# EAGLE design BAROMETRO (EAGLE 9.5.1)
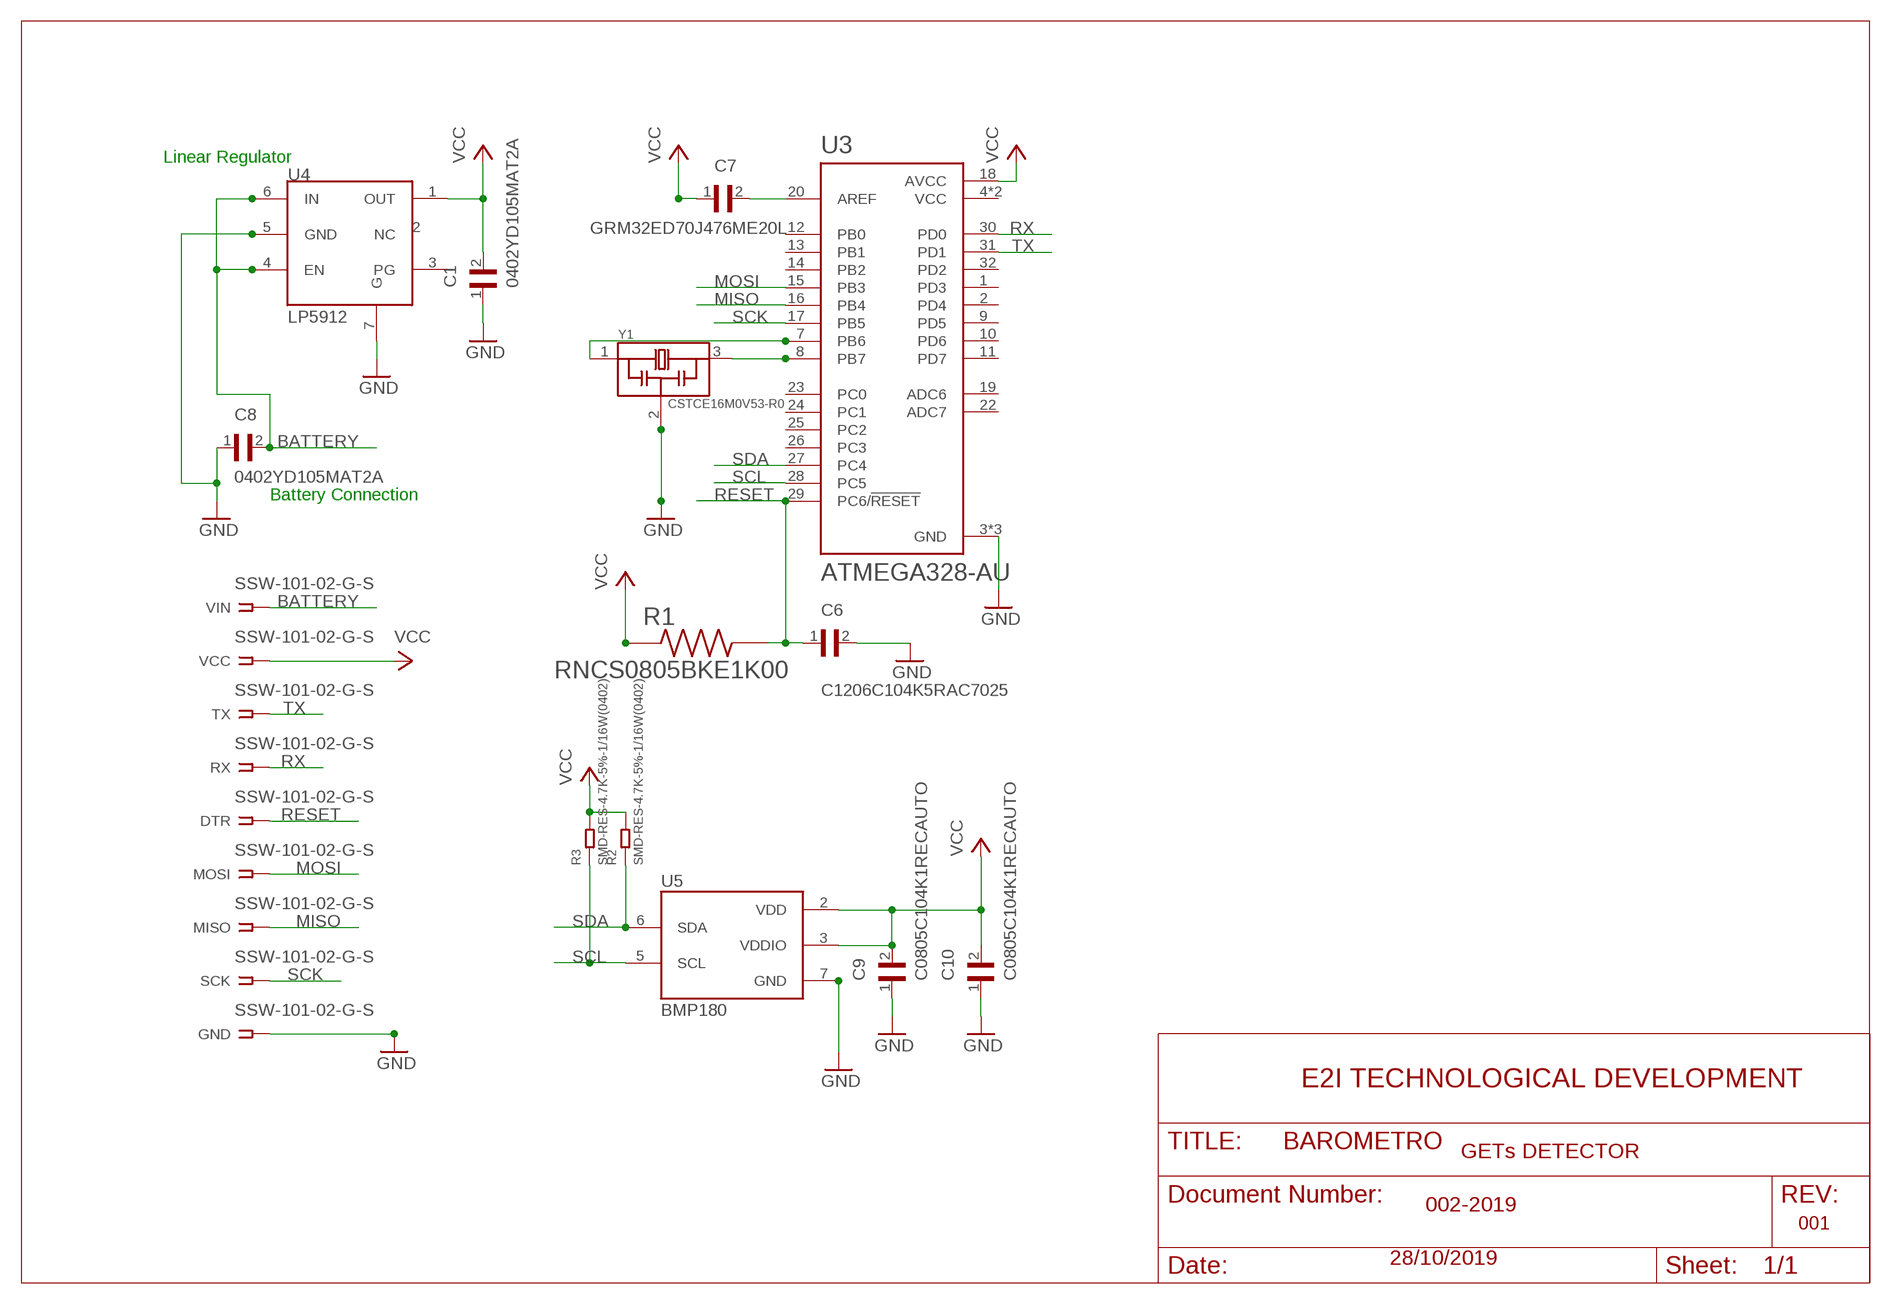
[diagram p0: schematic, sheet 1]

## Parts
C1  0402YD105MAT2A  [CAPC1005X71N]
C6  C1206C104K5RAC7025  [CAPC3216X88N]
C7  GRM32ED70J476ME20L  [CAPC3225X270N]
C8  0402YD105MAT2A  [CAPC1005X71N]
C9  C0805C104K1RECAUTO  [CAPC2012X110N]
C10  C0805C104K1RECAUTO  [CAPC2012X110N]
DTR  SSW-101-02-G-S  [SSW-101-02-G-S]
GND  SSW-101-02-G-S  [SSW-101-02-G-S]
MISO  SSW-101-02-G-S  [SSW-101-02-G-S]
MOSI  SSW-101-02-G-S  [SSW-101-02-G-S]
R1  RNCS0805BKE1K00  [RESC2012X65N]
R2  SMD-RES-4.7K-5%-1/16W(0402)  [R0402]
R3  SMD-RES-4.7K-5%-1/16W(0402)  [R0402]
RX  SSW-101-02-G-S  [SSW-101-02-G-S]
SCK  SSW-101-02-G-S  [SSW-101-02-G-S]
TX  SSW-101-02-G-S  [SSW-101-02-G-S]
U3  ATMEGA328-AU  [QFP80P900X900X120-32N]
U4  LP5912  [LP5912]
U5  BMP180  [BMP180]
VCC  SSW-101-02-G-S  [SSW-101-02-G-S]
VIN  SSW-101-02-G-S  [SSW-101-02-G-S]
Y1  CSTCE16M0V53-R0  [OSC_CSTCE16M0V53-R0]

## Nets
BATTERY: C8.2 U4.4(EN) U4.6(IN) VIN.1
GND: C1.1 C6.2 C8.1 C9.1 C10.1 GND.1 U3.3(GND) U3.5(GND) U3.21(GND) U4.5(GND) U4.7(G) U5.7(GND) Y1.2
MISO: MISO.1 U3.16(PB4)
MOSI: MOSI.1 U3.15(PB3)
N$1: U3.7(PB6) Y1.1
N$2: U3.8(PB7) Y1.3
N$11: C7.2 U3.20(AREF)
RESET: C6.1 DTR.1 R1.2 U3.29(PC6/!RESET)
RX: RX.1 U3.30(PD0)
SCK: SCK.1 U3.17(PB5)
SCL: R3.1 U3.28(PC5) U5.5(SCL)
SDA: R2.1 U3.27(PC4) U5.6(SDA)
TX: TX.1 U3.31(PD1)
VCC: C1.2 C7.1 C9.2 C10.2 R1.1 R2.2 R3.2 U3.18(AVCC) U4.1(OUT) U5.2(VDD) U5.3(VDDIO) VCC.1
Unconnected: U3.1(PD3) U3.2(PD4) U3.9(PD5) U3.10(PD6) U3.11(PD7) U3.12(PB0) U3.13(PB1) U3.14(PB2) U3.19(ADC6) U3.22(ADC7) U3.23(PC0) U3.24(PC1) U3.25(PC2) U3.26(PC3) U3.32(PD2) U4.2(NC) U4.3(PG)

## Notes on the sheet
- Linear Regulator
- Battery Connection
- E2I TECHNOLOGICAL DEVELOPMENT
- GETs DETECTOR
- 002-2019
- 001
- 28/10/2019

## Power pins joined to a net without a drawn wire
VCC: U3.4(VCC) U3.6(VCC)

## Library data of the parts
C1 C8 = Capacitor1uF:0402YD105MAT2A: CAP 1UF 16VDC X5R 20% SMD 0402; AVAILABILITY: Unavailable; DESCRIPTION: Cap 1uf 16vdc X5r 20% Smd 0402; MF: AVX; MP: 0402YD105MAT2A; PACKAGE: 1005 AVX; PRICE: None
C6 = Cap Ceramic 0.1uF smd:C1206C104K5RAC7025; AVAILABILITY: Unavailable; DESCRIPTION: Cap Ceramic 0.1uF 50V X7R 10% SMD 1206 125C Plastic T/R; MF: KEMET; MP: C1206C104K5RAC7025; PACKAGE: 3216 KEMET; PRICE: None
C7 = capacitor 47uF smd:GRM32ED70J476ME20L: CAP 47UF 6.3VDC X7T 20% SMD 1210 EMBOSSED TAPE; AVAILABILITY: Unavailable; DESCRIPTION: Cap 47uf 6.3vdc X7t 20% Smd 1210 Embossed Tape; MF: Murata; MP: GRM32ED70J476ME20L; PACKAGE: 1210 Murata; PRICE: None
C9 C10 = Capacitor smd 104K1-RECAUTO:C0805C104K1RECAUTO: Cap Ceramic 0.1uF 100V X7R 10% Pad SMD 0805 125C T/R; AVAILABILITY: Unavailable; DESCRIPTION: Capacitor: ceramic; MLCC; 100nF; 100V; X7R; ±10%; SMD; 0805; MF: KEMET; MP: C0805C104K1RECAUTO; PACKAGE: 2012 KEMET; PRICE: None
DTR GND MISO MOSI RX SCK TX VCC VIN = con-samtec:SSW-101-02-G-S: THROUGH-HOLE .025" SQ POST SOCKET; MF: Samtec Inc.; MPN: SSW-101-02-G-S; OC_FARNELL: unknown; OC_NEWARK: 11P9336
R1 = smd1kresistor:RNCS0805BKE1K00; AVAILABILITY: Unavailable; DESCRIPTION: Res Thin Film 0805 1K Ohm 0.1% 0.1W_1/10W_ ±25ppm/C Pad SMD T/R; MF: Stackpole Electronics Inc; MP: RNCS0805BKE1K00; PACKAGE: 2012 Stackpole; PRICE: None
R2 R3 = RES-4.7K-SMD-5_-1_16W_0402_:SMD-RES-4.7K-5%-1/16W(0402): 301010010; AVAILABILITY: Unavailable; DESCRIPTION: Res Thick Film 0402 4.7K Ohm 5% 0.063W_1/16W_ ?100ppm/C Molded SMD Paper T/R; MF: Yageo; MP: RC0402JR074K7L; PACKAGE: 0402 Yageo; PRICE: None
U3 = ATMEGA328-AU:ATMEGA328-AU: ATmega Series 20 MHz 32 KB Flash 2 KB SRAM 8-Bit Microcontroller - TQFP-32; AVAILABILITY: Unavailable; DESCRIPTION: ATmega Series 20 MHz 32 KB Flash 2 KB SRAM 8-Bit Microcontroller - TQFP-32; MF: Microchip; MP: ATMEGA328-AU; PACKAGE: TQFP-32 Microchip; PRICE: None
U4 = electronic-labs:LP5912
U5 = BMP180:BMP180: BOSCH BMP180 DIGITAL BAROMETRIC PRESSURE SENSOR Web page: http://www.bosch-sensortec.com/en/homepage/products_3/environmental_sensors_1/bmp180_1/bmp180 Datasheet: http://ae-bst.resource.bosch.com/media/products/dokumente/bmp180/BST-BMP180-DS000-09.pdf The BMP180 is the function compatible successor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; AVAILABILITY: Unavailable; DESCRIPTION: Sensor Pressure Abs; MF: Bosch Sensortec; MP: BMP180; PACKAGE: VLGA-7 Bosch Sensortec; PRICE: None
Y1 = CSTCE16M0V53-R0:CSTCE16M0V53-R0: 16MHz Ceramic Resonator Built in Capacitor 15pF ±0.3% -20°C ~ 80°C Surface Mount; AVAILABILITY: Unavailable; DESCRIPTION: Ceramic Resonator 16MHz ??0.5% _Tol_ ??0.3% _Stability_ 15pF 40Ohm 3-Pin CSMD T/R; MF: Murata; MP: CSTCE16M0V53-R0; PACKAGE: SMD-3 Murata; PRICE: None

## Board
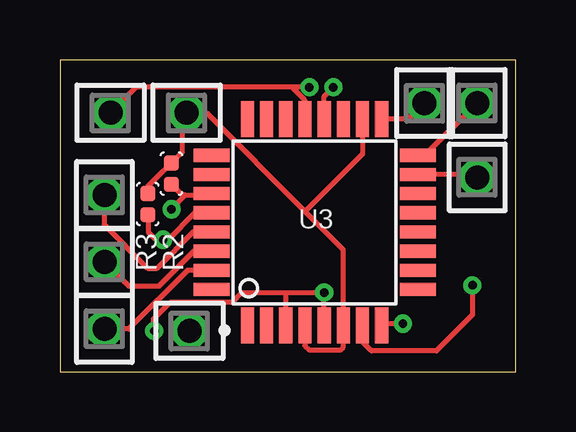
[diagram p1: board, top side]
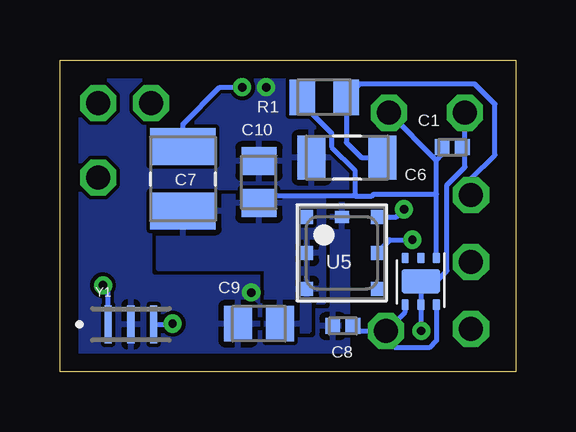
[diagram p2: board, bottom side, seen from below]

Size 19 x 13 mm. Coordinates in mm from the lower left corner, seen from the top.
Outline: 19,0 19,13 0,13 0,0 19,0
Copper layers (1*16): Top 0.035mm / dielectric 1.5mm / Bottom 0.035mm
Design rules "default *": minimum track width 6mil, minimum drill 0.35mm, track to track 6mil, track to pad 6mil, pad to pad 6mil, via to via 6mil, smd to smd 6mil, copper to edge 30mil, drill to drill 6mil, minimum pad ring 10mil, minimum via ring 8mil, stop-mask expansion 4mil, vias tented up to drill 0.5mm, thermal gap 10mil

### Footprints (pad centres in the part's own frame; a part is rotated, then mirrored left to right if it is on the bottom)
CAPC1005X71N = smd 0.62 x 0.67: 1 -0.425,0; 2 0.425,0
CAPC3216X88N = smd 1.16 x 1.82: 1 -1.475,0; 2 1.475,0
CAPC3225X270N = smd 1.53 x 2.72: 1 -1.341,0; 2 1.341,0
CAPC2012X110N = smd 1.16 x 1.47: 1 -0.875,0; 2 0.875,0
SSW-101-02-G-S = drill 1 pad 1.5 octagon: 1 0,0
RESC2012X65N = smd 1.06 x 1.47: 1 -0.925,0; 2 0.925,0
R0402 = smd 0.635 x 0.635: 1 0,0.445; 2 0,-0.445
QFP80P900X900X120-32N = smd 1.5 x 0.55: 1 -4.3,2.8; 2 -4.3,2; 3 -4.3,1.2; 4 -4.3,0.4; 5 -4.3,-0.4; 6 -4.3,-1.2; 7 -4.3,-2; 8 -4.3,-2.8; 17 4.3,-2.8; 18 4.3,-2; 19 4.3,-1.2; 20 4.3,-0.4; 21 4.3,0.4; 22 4.3,1.2; 23 4.3,2; 24 4.3,2.8 | smd 0.55 x 1.5: 9 -2.8,-4.3; 10 -2,-4.3; 11 -1.2,-4.3; 12 -0.4,-4.3; 13 0.4,-4.3; 14 1.2,-4.3; 15 2,-4.3; 16 2.8,-4.3; 25 2.8,4.3; 26 2,4.3; 27 1.2,4.3; 28 0.4,4.3; 29 -0.4,4.3; 30 -1.2,4.3; 31 -2,4.3; 32 -2.8,4.3
LP5912 = smd 0.45 x 0.3: 1 0,0.65; 2 0,0; 3 0,-0.65; 4 1.95,-0.65; 5 1.95,0; 6 1.95,0.65 | smd 1 x 1.6: 7 0.975,0
BMP180 = smd 0.6 x 0.5: 1 1.5,1.45; 2 0,1.45; 3 -1.5,1.45; 4 -1.5,-1.45; 5 0,-1.45; 6 1.5,-1.45 | smd 0.5 x 0.6: 7 1.5,0
OSC_CSTCE16M0V53-R0 = smd 0.3 x 1.6: 1 -0.95,0; 2 0,0; 3 0.95,0

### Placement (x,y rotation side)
C1  2.64,9.36 180 bottom
C6  7.03,8.93 180 bottom
C7  13.87,8.04 90 bottom
C8  7.2,1.9 0 bottom
C9  10.7,2 0 bottom
C10  10.7,7.9 270 bottom
DTR  1.85,7.37 90 top
GND  2.11,10.79 180 top
MISO  17.4,11.2 90 top
MOSI  17.4,8.1 90 top
R1  7.98,11.44 0 bottom
R2  4.65,8.26 180 top
R3  3.66,6.98 180 top
RX  1.85,4.57 90 top
SCK  15.2,11.2 270 top
TX  1.85,1.78 90 top
U3  10.62,6.22 90 top
U4  3.95,4.74 270 bottom
U5  7.24,4.95 90 bottom
VCC  5.28,10.79 180 top
VIN  5.4,1.7 180 top
Y1  16.04,1.97 0 bottom

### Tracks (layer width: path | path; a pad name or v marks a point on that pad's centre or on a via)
BATTERY
  Bottom 0.2: C8.2 6.57,1.7 VIN.1 | VIN.1 4.6,2.5 U4.4 | U4.6 3.3,1.3 3.6,1 5,1 5.4,1.4 VIN.1
GND  (via drill 0.35)
  Top 0.2: GND.1 3.2,11.88 9.66,11.88 | U3.21 10.22,11.32 9.66,11.88 | U3.5 v11.02,3.3 9.4,3.3 | 9.66,11.88 10.38,11.88 v10.4,11.86 | v3.93,1.7 3.9,1.73 3.9,2.2 4.6,2.9 7.2,2.9 7.6,3.3 9.4,3.3 | U3.3 9.42,3.28 9.4,3.3
  Bottom 0.2: 2.11,9.3 2.11,8.54 2.86,7.78 2.86,4.2 3.3,3.77 U4.7 U4.5 3.95,1.72 v3.93,1.7 | 2.11,9.3 GND.1 | C1.1 2.15,9.3 2.11,9.3
  pour Bottom (rank 6): 7,0.1 7,12.8 18.8,12.8 18.8,0.1
MISO
  Top 0.2: U3.16 15.22,9.02 MISO.1
MOSI
  Top 0.2: MOSI.1 17.28,8.22 U3.15
N$1  (via drill 0.35)
  Top 0.2: U3.7 12.6,1.91 12.6,1.26 13,0.86 15.7,0.86 17.2,2.36 v17.2,3.6
  Bottom 0.2: Y1.1 16.99,3.39 v17.2,3.6
N$2  (via drill 0.35)
  Top 0.2: v14.3,2 13.5,2 U3.8
  Bottom 0.2: Y1.3 14.33,1.97 v14.3,2
N$11  (via drill 0.35)
  Top 0.2: U3.20 11.02,11.48 v11.4,11.86
  Bottom 0.2: v11.4,11.86 12.34,11.86 13.87,10.33 C7.2
RESET
  Top 0.2: U3.29 5.56,5.82 4.02,4.29 3.68,4.29 1.85,6.11 DTR.1
  Bottom 0.2: DTR.1 1.85,8.04 0.86,9.04 0.86,11.16 1.7,12 6.49,12 R1.2 7.05,9.55 6.43,8.93 C6.1
RX
  Top 0.2: U3.30 5.59,5.02 4.14,3.57 2.85,3.57 RX.1
SCK
  Top 0.2: SCK.1 14.52,10.52 U3.17
SCL  (via drill 0.35)
  Top 0.2: U3.28 5.62,6.62 4.5,5.5 v4.3,5.5 4,5.5 3.7,5.8 3.7,6.5 R3.1
  Bottom 0.2: U5.5 5.24,5.5 v4.3,5.5
SDA  (via drill 0.35)
  Top 0.2: v4.65,6.77 5.24,7.36 | 5.24,7.36 6.25,7.36 U3.27 | 5.24,7.36 5.1,7.36 R2.1
  Bottom 0.2: U5.6 4.97,6.45 v4.65,6.77
TX
  Top 0.2: U3.31 5.32,4.22 2.87,1.78 TX.1
VCC
  Top 0.2: R3.2 3.66,7.72 4.32,8.38 4.33,8.38 R2.2 5.1,9.15 5.1,10.61 VCC.1 6.11,10.79 10.22,6.68 | U3.18 12.62,9.08 10.22,6.68 | U3.4 10.22,1.08 10.4,0.9 11.7,0.9 11.82,1.02 U3.6 11.82,5.08 10.22,6.68
  Bottom 0.2: R1.1 8.9,11.18 7.67,9.95 7.67,9.37 6.7,8.4 6.7,7.32 | 6.7,7.32 10.4,7.32 C10.2 | U4.1 3.3,7.4 | 3.3,7.4 3.3,8.81 | VCC.1 3.3,8.81 | 3.3,8.81 3.06,9.05 C1.2 | 6.7,7.32 5.99,7.32 5.91,7.4 3.3,7.4 | 3.3,7.4
  pour Bottom (rank 3): 8,2.9 8,7.3 14.9,7.3 14.9,4.3 10.4,4.3 10.4,1.7 8.6,1.7 8.6,2.9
